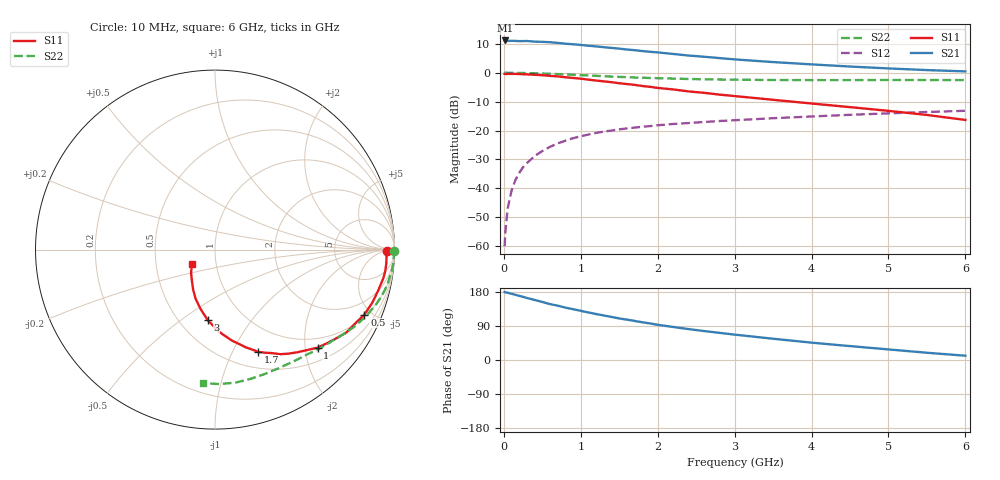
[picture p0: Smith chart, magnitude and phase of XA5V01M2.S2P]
! SIEMENS Discrete & RF Semiconductors
! BFY180
! Si NPN RF Bipolar Junction Transistor in MICRO-X
! VCE = 5 V  IC = 1.2 mA
! Common Emitter S-Parameters:  May  1997
# GHz  S  MA  R  50
!  f  S11  S21  S12  S22
! GHz  MAG  ANG  MAG  ANG  MAG  ANG  MAG  ANG
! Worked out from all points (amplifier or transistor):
!   36 points, 10 MHz to 6 GHz, reference 50 ohm
!   highest |S21| = 11.2 dB at 20 MHz (marker M1)
!   |S21| within 3 dB of that: start of sweep to 1.556 GHz
!   unconditionally stable (mu >= 1): 3.754 GHz to end of sweep
!   at 250 MHz: K = 0.08, MSG = 21.8 dB, |S12| = -32.7 dB
!   at 1.4 GHz: K = 0.53, MSG = 14.3 dB, |S12| = -20.0 dB
!   at 6 GHz: K = 1.05, MAG = 5.4 dB, |S12| = -13.2 dB
!   S11 on the Smith chart (normalised r, x): 10 MHz: 43, -8; 500 MHz: 1.11, -4.55; 1 GHz: 0.78, -2.27; 1.7 GHz: 0.69, -1.26; 3 GHz: 0.68, -0.64; 6 GHz: 0.76, -0.13
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0.01  0.9565 -0.5  3.585 179.2  0.001 88.0  0.9984 -0.3
0.02  0.9502 -0.7  3.624 178.6  0.0018 83.6  0.9999 -0.5
0.05  0.9567 -2.3  3.545 177.4  0.0045 86.7  0.9978 -1.4
0.1  0.9574 -4.8  3.58 174.8  0.0091 88.3  0.9972 -2.8
0.15  0.9563 -7.1  3.556 172.1  0.0139 85.6  0.9968 -4.1
0.25  0.9431 -12.0  3.535 166.8  0.0233 82.6  0.9917 -7.0
0.3  0.9375 -14.1  3.544 163.7  0.0274 81.1  0.9868 -8.3
0.5  0.9072 -23.5  3.43 153.1  0.0443 73.8  0.9722 -13.6
0.6  0.8826 -27.9  3.379 147.5  0.0523 71.1  0.9609 -16.1
0.8  0.837 -36.2  3.184 138.3  0.0667 65.6  0.935 -20.9
1  0.7906 -43.7  3.029 129.7  0.0797 60.2  0.9102 -25.2
1.1  0.76 -47.4  2.938 125.5  0.0854 57.9  0.8976 -27.1
1.4  0.6872 -58.0  2.691 113.6  0.1001 51.9  0.8597 -32.9
1.7  0.6184 -67.1  2.459 103.1  0.1127 47.3  0.8282 -37.8
2  0.5467 -75.2  2.251 92.9  0.1236 43.2  0.8066 -42.3
2.2  0.5154 -79.5  2.117 87.2  0.1299 40.8  0.7942 -45.3
2.6  0.4504 -88.3  1.896 76.5  0.1407 36.8  0.7719 -50.5
3  0.3955 -95.8  1.704 67.0  0.1511 33.2  0.7592 -55.6
3.5  0.3407 -103.6  1.532 56.1  0.1636 29.4  0.7501 -61.7
4.5  0.2544 -118.6  1.282 36.7  0.1874 21.9  0.747 -74.6
5.5  0.1863 -135.7  1.113 19.1  0.2096 14.3  0.7493 -88.2
6  0.1527 -147.5  1.057 11.3  0.22 10.2  0.7475 -95.1
